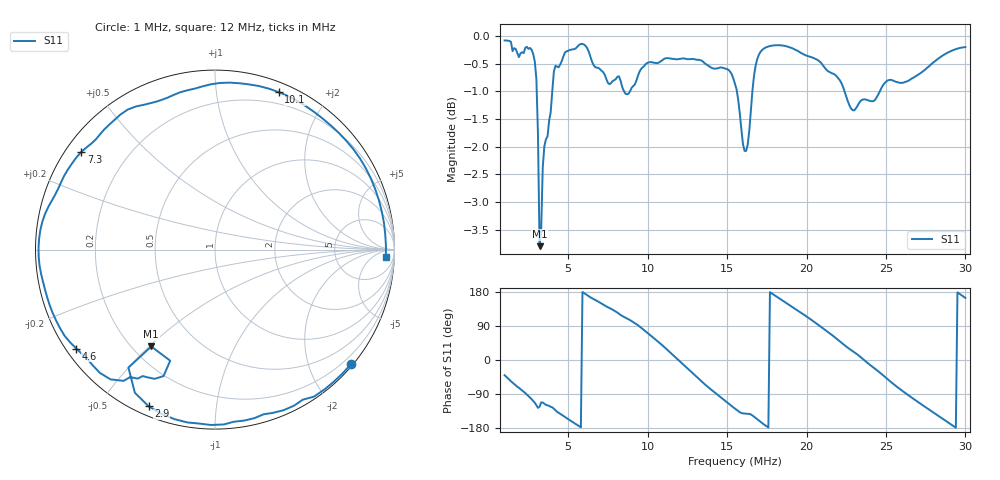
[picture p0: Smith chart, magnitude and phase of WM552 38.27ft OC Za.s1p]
!Created via Zplots "Save as S1P" button
!Original data file:  $remote$.s1p
!Transmission line transform:  None
# MHZ S MA R 400
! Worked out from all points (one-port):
!   291 points, 1 MHz to 30 MHz, reference 400 ohm
!   lowest |S11| = -3.8 dB at 3.2 MHz (marker M1), VSWR 4.65, Z = 110 - j203 ohm
!   |S11| at or under -10 dB: nowhere
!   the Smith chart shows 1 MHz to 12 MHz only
!   S11 on the Smith chart (normalised r, x): 1 MHz: 0.04, -2.73; 2.9 MHz: 0.04, -0.66; 4.6 MHz: 0.03, -0.32; 7.3 MHz: 0.04, +0.33; 10.1 MHz: 0.09, +1.48; 12 MHz: 22, -21
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1  0.9904 -40.2
2.1  0.9664 -80.2
2.9  0.9481 -113.0
3.1  0.8152 -126.3
3.2  0.646 -123.3
3.3  0.6674 -112.0
4  0.8914 -124.9
4.6  0.9491 -144.5
4.7  0.9581 -147.3
5.9  0.9832 179.5
7.3  0.9225 143.8
8.3  0.9109 118.8
10.1  0.9466 67.9
11.9  0.9526 1.4
12  0.953 -2.6
13.7  0.9424 -67.8
14.6  0.9364 -98.2
15.5  0.9049 -128.3
16.7  0.9212 -149.7
17.5  0.977 -175.3
19.2  0.9731 137.3
21  0.942 84.8
22.8  0.86 26.4
24.6  0.8901 -32.6
25.5  0.9104 -64.4
26.4  0.9108 -92.6
28.4  0.9563 -150.2
30  0.9767 163.9
